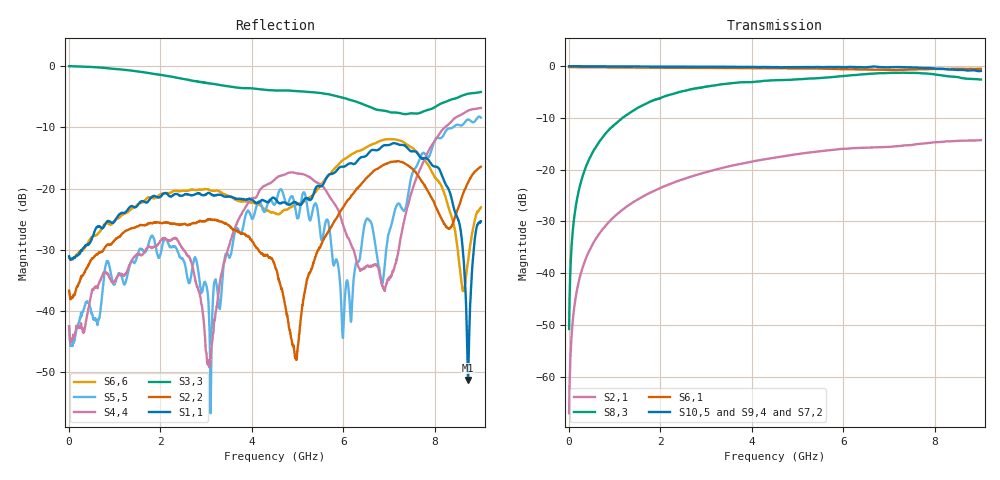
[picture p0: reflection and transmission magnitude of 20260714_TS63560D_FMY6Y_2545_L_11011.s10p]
# GHz S DB R 50
! CMT, SN0916, 25263762, 26.7.0
! Date: 15.07.2026 13:49:11
! Data: Format
! Freq S1.1:dB/Ang S1.2:dB/Ang S1.3:dB/Ang S1.4:dB/Ang S1.5:dB/Ang S1.6:dB/Ang S1.7:dB/Ang S1.8:dB/Ang S1.9:dB/Ang S1.10:dB/Ang
!  S2.1:dB/Ang S2.2:dB/Ang S2.3:dB/Ang S2.4:dB/Ang S2.5:dB/Ang S2.6:dB/Ang S2.7:dB/Ang S2.8:dB/Ang S2.9:dB/Ang S2.10:dB/Ang
!  S3.1:dB/Ang S3.2:dB/Ang S3.3:dB/Ang S3.4:dB/Ang S3.5:dB/Ang S3.6:dB/Ang S3.7:dB/Ang S3.8:dB/Ang S3.9:dB/Ang S3.10:dB/Ang
!  S4.1:dB/Ang S4.2:dB/Ang S4.3:dB/Ang S4.4:dB/Ang S4.5:dB/Ang S4.6:dB/Ang S4.7:dB/Ang S4.8:dB/Ang S4.9:dB/Ang S4.10:dB/Ang
!  S5.1:dB/Ang S5.2:dB/Ang S5.3:dB/Ang S5.4:dB/Ang S5.5:dB/Ang S5.6:dB/Ang S5.7:dB/Ang S5.8:dB/Ang S5.9:dB/Ang S5.10:dB/Ang
!  S6.1:dB/Ang S6.2:dB/Ang S6.3:dB/Ang S6.4:dB/Ang S6.5:dB/Ang S6.6:dB/Ang S6.7:dB/Ang S6.8:dB/Ang S6.9:dB/Ang S6.10:dB/Ang
!  S7.1:dB/Ang S7.2:dB/Ang S7.3:dB/Ang S7.4:dB/Ang S7.5:dB/Ang S7.6:dB/Ang S7.7:dB/Ang S7.8:dB/Ang S7.9:dB/Ang S7.10:dB/Ang
!  S8.1:dB/Ang S8.2:dB/Ang S8.3:dB/Ang S8.4:dB/Ang S8.5:dB/Ang S8.6:dB/Ang S8.7:dB/Ang S8.8:dB/Ang S8.9:dB/Ang S8.10:dB/Ang
!  S9.1:dB/Ang S9.2:dB/Ang S9.3:dB/Ang S9.4:dB/Ang S9.5:dB/Ang S9.6:dB/Ang S9.7:dB/Ang S9.8:dB/Ang S9.9:dB/Ang S9.10:dB/Ang
!  S10.1:dB/Ang S10.2:dB/Ang S10.3:dB/Ang S10.4:dB/Ang S10.5:dB/Ang S10.6:dB/Ang S10.7:dB/Ang S10.8:dB/Ang S10.9:dB/Ang S10.10:dB/Ang
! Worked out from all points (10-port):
!   2001 points, 10 MHz to 9 GHz, reference 50 ohm
!   strongest paths, dB at 10 MHz, 2.257 GHz, 4.505 GHz, 6.753 GHz, 9 GHz:
!     S10,5: -0.1, -0.2, -0.2, -0.2, -1.0
!     S9,4: -0.1, -0.2, -0.4, -0.4, -1.5
!     S7,2: -0.1, -0.3, -0.4, -0.6, -0.6
!     S6,1: -0.3, -0.4, -0.5, -0.7, -0.6
!     S8,3: -50.7, -5.5, -2.8, -1.4, -2.6
!     S2,1: -67.0, -22.6, -17.7, -15.7, -14.3
!   lowest |S11| = -51.3 dB at 8.721 GHz (marker M1), VSWR 1.01, Z = 49.9 + j0.246 ohm
!   |S11| at or under -10 dB: start of sweep to end of sweep
